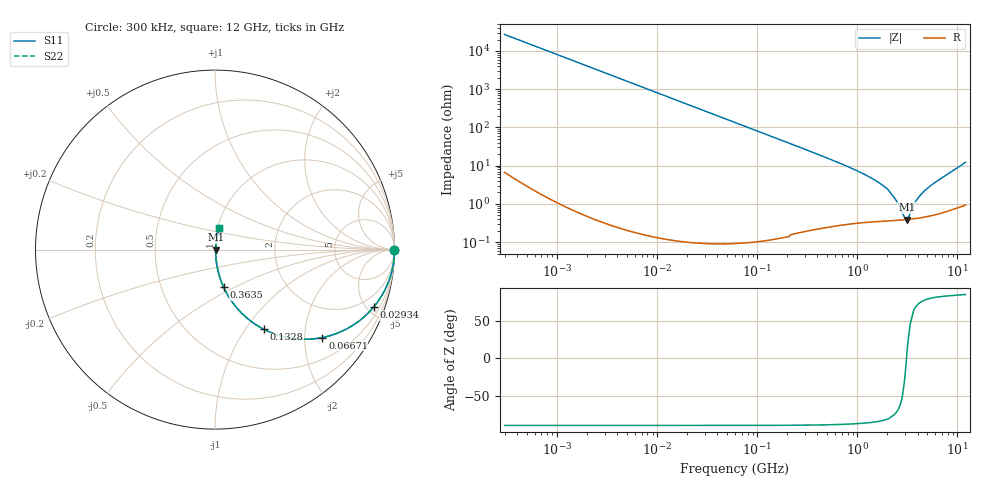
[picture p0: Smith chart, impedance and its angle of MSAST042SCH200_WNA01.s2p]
! MSAST042SCH200_WNA01  S-PARAMETER MODEL  ( General Type )
! Model Generated by TAIYO YUDEN Corporation (http://www.ty-top.com)
! Version 1.0
! TAIYO YUDEN Control No. 150820
! Copyright(c) 2015 TAIYO YUDEN CO.,LTD. All Rights Reserved.
! Product Description (link to TY-COMPAS)
! https://ds.yuden.co.jp/TYCOMPAS/or/detail?pn=MSAST042SCH200JWNA01&u=M
! Products Name : Multilayer Ceramic Capacitors
! Characteristics :
!  Capacitance : 20 pF , Rated Voltage : 25V , TCC : CH / C0H
!  Case Size : 0.4 x 0.2 / 0.016 x 0.008 [mm/inch] , Thickness : 0.2 / 0.008 [mm/inch]
!  (Conditions: Temperature = 25 degC , DC Bias Current/Voltage = 0A / 0V)
! External Node Assignments :
!  1  o---| |---o  2
! GND o---------o GND
! Frequency Range : 0.3MHz  -  12000MHz  [ 401 STEP ]
# MHz S RI R 50
! Freq[MHz].  S11 Real  S11 Imag  S21 Real  S21 Imag  S12 Real  S12 Imag  S22 Real  S22 Imag
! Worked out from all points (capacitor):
!   401 points, 300 kHz to 12 GHz, reference 50 ohm
!   read as one part in series: C = 19.6 pF near 316.3 kHz
!   lowest |Z| = 390 mohm at 3.108 GHz (marker M1)
!   series resonance near 3.097 GHz, so ESL is about 140 pH
!   S11 on the Smith chart (normalised r, x): 300 kHz: open; 29.34 MHz: 1.00, -5.55; 66.71 MHz: 1.00, -2.44; 132.8 MHz: 1.00, -1.22; 363.5 MHz: 1.00, -0.44; 12 GHz: 1.02, +0.24
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0.3  1 -0.00369  1.45e-05 0.00369  1.45e-05 0.00369  1 -0.00369
1.769972  0.9995 -0.0217  0.000475 0.0217  0.000475 0.0217  0.9995 -0.0217
10.44266  0.9838 -0.1262  0.0162 0.1262  0.0162 0.1262  0.9838 -0.1262
29.34352  0.8849 -0.319  0.1151 0.319  0.1151 0.319  0.8849 -0.319
60  0.6477 -0.4773  0.3523 0.4773  0.3523 0.4773  0.6477 -0.4773
66.70707  0.598 -0.4899  0.402 0.4899  0.402 0.4899  0.598 -0.4899
91.67136  0.4405 -0.4959  0.5595 0.4959  0.5595 0.4959  0.4405 -0.4959
132.8329  0.2727 -0.4444  0.7273 0.4444  0.7273 0.4444  0.2727 -0.4444
208.3979  0.1323 -0.337  0.8677 0.337  0.8677 0.337  0.1323 -0.337
353.9943  0.0508 -0.215  0.9492 0.215  0.9492 0.215  0.0508 -0.215
363.4975  0.0483 -0.2098  0.9517 0.2098  0.9517 0.2098  0.0483 -0.2098
1197.383  0.00658 -0.0574  0.9934 0.0574  0.9934 0.0574  0.00658 -0.0574
1689.663  0.00463 -0.0338  0.9954 0.0338  0.9954 0.0338  0.00463 -0.0338
2088.533  0.00403 -0.0208  0.996 0.0208  0.996 0.0208  0.00403 -0.0208
2514.07  0.00382 -0.0102  0.9962 0.0102  0.9962 0.0102  0.00382 -0.0102
2947.191  0.00384 -0.00236  0.9962 0.00236  0.9962 0.00236  0.00384 -0.00236
3107.553  0.00388 0.000165  0.9961 -0.000165  0.9961 -0.000165  0.00388 0.000165
3276.641  0.00394 0.00256  0.9961 -0.00256  0.9961 -0.00256  0.00394 0.00256
3944.255  0.00433 0.0122  0.9957 -0.0122  0.9957 -0.0122  0.00433 0.0122
4747.894  0.00501 0.022  0.995 -0.022  0.995 -0.022  0.00501 0.022
6354.153  0.00697 0.04  0.993 -0.04  0.993 -0.04  0.00697 0.04
12000  0.0235 0.118  0.9765 -0.118  0.9765 -0.118  0.0235 0.118
